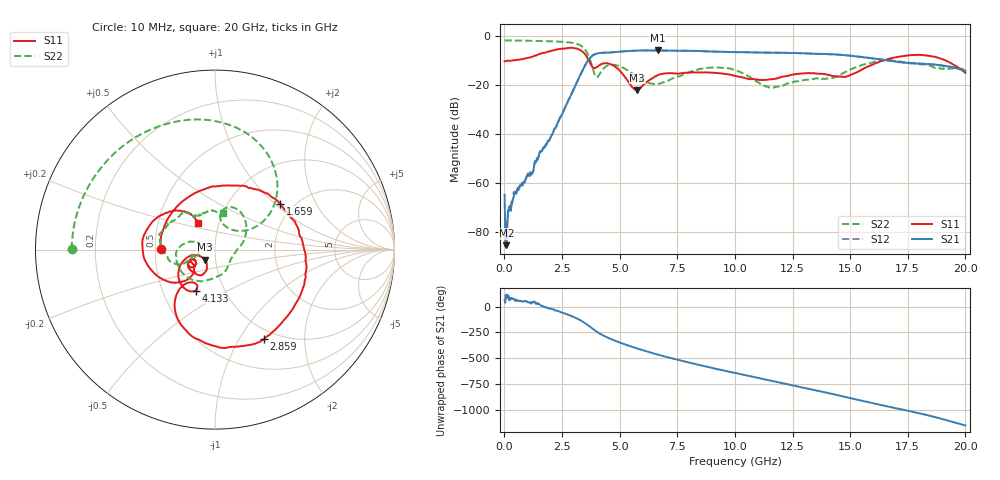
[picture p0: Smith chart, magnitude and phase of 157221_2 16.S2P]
!  2-Port S-parameters saved by WinCal
! VAR MeasName=S-Parameters (CALIBRATED_DATA) read from VNA (N5242A)
! VAR MeasDate=2015-5-26 16:48:09
! VAR NAME=157221_2 16
! VAR FILENAME=157221_2 16.S2P
! VAR DATE=2015-5-26 16:48:10
! VAR PHYS_PORTS=1,2
# Hz S DB R 50
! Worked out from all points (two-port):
!   801 points, 10 MHz to 20 GHz, reference 50 ohm
!   highest |S21| = -6.01 dB at 6.657 GHz (marker M1); lowest = -85.3 dB at 84.96 MHz (marker M2)
!   |S21| within 3 dB of the highest: 3.723 GHz to 15.77 GHz (12.05 GHz wide, 124 % of centre)
!   lowest |S11| = -22.1 dB at 5.757 GHz (marker M3), VSWR 1.17, Z = 44.5 - j4.99 ohm
!   |S11| at or under -10 dB: start of sweep to 443.2 MHz; 3.658 GHz to 16.48 GHz (12.82 GHz wide, 127 % of centre); 19.13 GHz to end of sweep
!   |S22| runs from -21.2 to -2.0 dB; largest |S21 - S12| = 0.0083
!   S11 on the Smith chart (normalised r, x): 10 MHz: 0.54, +0.00; 1.659 GHz: 1.70, +1.08; 2.859 GHz: 0.87, -1.28; 4.133 GHz: 0.73, -0.36; 20 GHz: 0.79, +0.24
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1e7  -10.43 179.4  -64.78 64.8  -80.70 -112.6  -1.96 179.8
8.49625e7  -10.31 172.8  -85.30 84.7  -80.94 68.7  -1.96 177.8
4.847625e8  -9.98 136.0  -64.00 54.4  -64.01 56.4  -1.99 168.3
1.659175e9  -7.06 35.3  -46.25 4.9  -46.33 5.2  -2.18 138.2
2.283862e9  -5.65 -15.2  -36.11 -38.8  -36.10 -38.6  -2.39 118.5
2.858575e9  -4.89 -61.5  -24.73 -86.8  -24.67 -86.8  -2.79 94.3
3.358325e9  -6.27 -108.1  -14.76 -140.2  -14.70 -140.5  -4.33 61.2
3.758125e9  -11.83 -131.1  -8.66 156.4  -8.65 156.1  -10.93 29.5
4.132938e9  -11.95 -115.4  -7.08 98.4  -7.06 98.2  -15.61 78.5
4.932538e9  -13.57 -156.1  -6.59 17.7  -6.57 17.4  -12.23 49.4
5.757125e9  -22.08 -134.8  -6.09 -46.6  -6.09 -47.0  -16.75 8.9
6.656675e9  -16.10 -116.4  -6.01 -106.3  -6.00 -106.4  -19.67 -33.4
6.681662e9  -15.95 -116.9  -6.02 -107.9  -5.99 -108.1  -19.61 -34.2
8.080962e9  -15.01 -138.3  -6.16 172.3  -6.15 172.0  -14.69 -108.7
9.055475e9  -15.08 -149.3  -6.49 121.7  -6.48 121.4  -12.97 -150.7
1.0005e10  -16.34 -157.1  -6.69 75.5  -6.69 75.1  -14.02 176.6
1.165418e10  -17.72 -142.8  -6.94 -3.3  -6.91 -3.7  -21.08 177.0
1.335332e10  -15.28 -150.5  -7.35 -85.4  -7.30 -85.7  -17.78 -167.2
1.497751e10  -16.15 -138.5  -8.15 -167.5  -8.13 -167.9  -13.90 -156.4
1.667666e10  -9.46 -151.0  -10.18 107.1  -10.17 107.0  -9.89 164.4
1.847576e10  -8.30 157.9  -11.64 18.0  -11.70 16.9  -12.30 126.1
2e10  -15.11 123.3  -14.32 -75.0  -14.33 -76.1  -13.72 78.1
